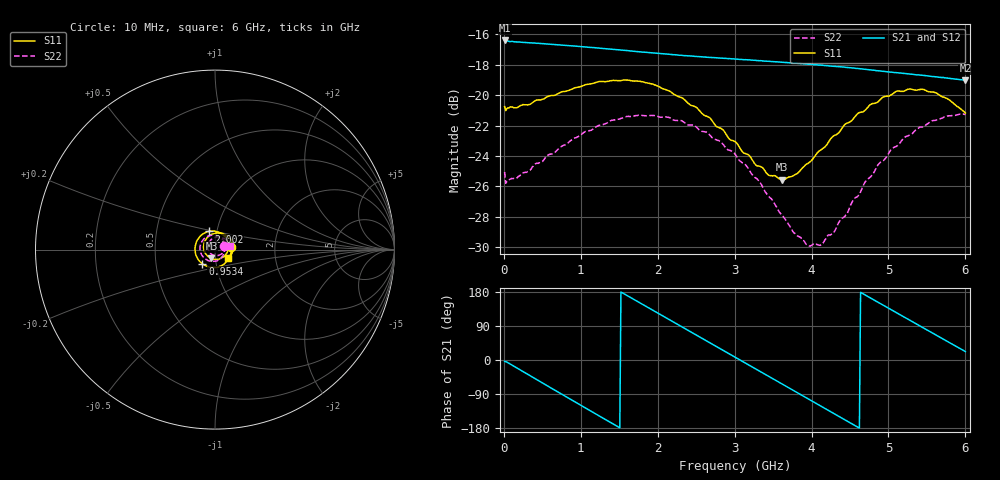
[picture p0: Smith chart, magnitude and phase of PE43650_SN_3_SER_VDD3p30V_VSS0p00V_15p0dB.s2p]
!Keysight Technologies,N5245B,MY57181451,A.13.50.07
!Date: Tuesday, May 07, 2019 08:00:15
!Correction: S11(Full 2 Port(1,2))
!S21(Full 2 Port(1,2))
!S12(Full 2 Port(1,2))
!S22(Full 2 Port(1,2))
!S2P File: Measurements: S11, S21, S12, S22:
# Hz S  dB  R 50
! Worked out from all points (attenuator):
!   401 points, 10 MHz to 6 GHz, reference 50 ohm
!   highest |S21| = -16.41 dB at 10 MHz (marker M1); lowest = -19.0 dB at 6 GHz (marker M2)
!   lowest |S11| = -25.6 dB at 3.619 GHz (marker M3), VSWR 1.11, Z = 47.8 - j4.69 ohm
!   |S11| at or under -10 dB: start of sweep to end of sweep
!   |S22| runs from -29.9 to -21.2 dB; largest |S21 - S12| = 0.0015
!   S11 on the Smith chart (normalised r, x): 10 MHz: 1.20, +0.04; 953.4 MHz: 0.86, -0.14; 2.002 GHz: 0.91, +0.19; 6 GHz: 1.16, -0.11
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1e7  -20.76 9.2  -16.41 -3.7  -16.44 -3.1  -25.05 20.0
1.44775e8  -20.83 -21.1  -16.50 -18.0  -16.56 -17.9  -25.49 -19.7
4.74225e8  -20.33 -68.5  -16.61 -57.3  -16.65 -57.3  -24.45 -66.8
7.13825e8  -19.88 -100.9  -16.70 -85.6  -16.76 -85.6  -23.51 -97.6
9.53425e8  -19.49 -131.1  -16.80 -113.9  -16.85 -114.0  -22.76 -125.3
1.013325e9  -19.42 -138.7  -16.83 -121.0  -16.87 -121.0  -22.57 -132.2
1.492525e9  -19.05 165.5  -17.03 -177.2  -17.09 -177.1  -21.59 178.2
1.732125e9  -19.08 138.6  -17.15 154.9  -17.20 154.8  -21.35 154.6
2.001675e9  -19.41 109.1  -17.26 123.6  -17.31 123.6  -21.41 128.9
2.01665e9  -19.44 107.4  -17.26 121.9  -17.32 121.9  -21.43 127.4
2.4659e9  -20.72 56.0  -17.44 69.9  -17.50 69.9  -21.98 84.1
3.005e9  -23.05 -12.1  -17.63 7.5  -17.69 7.6  -23.88 29.9
3.289525e9  -24.65 -55.1  -17.73 -25.3  -17.78 -25.3  -25.49 -3.4
3.618975e9  -25.56 -112.0  -17.85 -63.4  -17.89 -63.4  -27.91 -47.4
3.7837e9  -25.23 -141.5  -17.90 -82.6  -17.95 -82.5  -29.09 -73.9
4.008325e9  -24.25 -178.5  -17.98 -108.5  -18.03 -108.6  -29.84 -115.9
4.128125e9  -23.58 164.4  -18.04 -122.5  -18.09 -122.4  -29.83 -139.0
4.277875e9  -22.71 143.6  -18.10 -139.8  -18.15 -139.8  -29.08 -166.1
4.517475e9  -21.70 113.0  -18.21 -167.6  -18.26 -167.4  -27.12 155.4
5.01165e9  -20.05 59.2  -18.48 135.5  -18.53 135.6  -23.74 97.8
5.475875e9  -19.67 14.6  -18.72 82.2  -18.78 82.3  -22.02 54.6
6e9  -21.18 -31.4  -19.03 22.3  -19.07 22.4  -21.28 12.5
